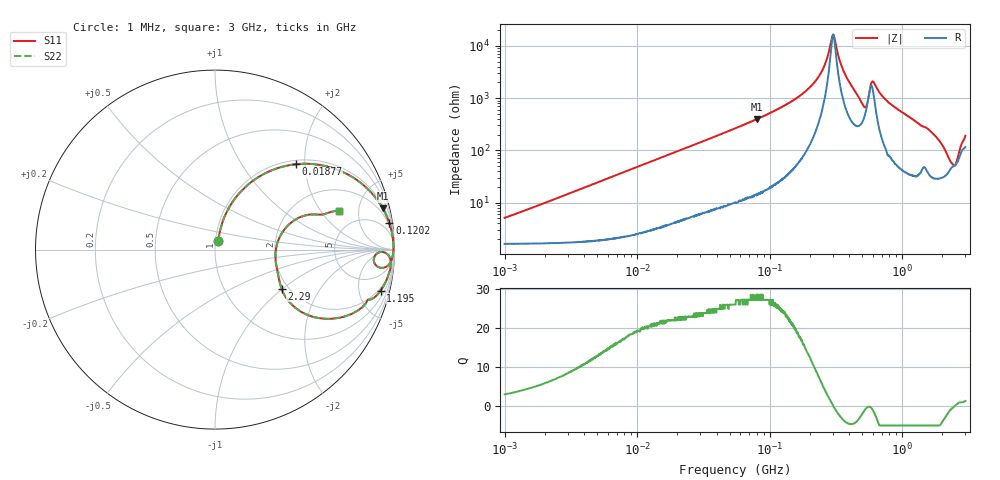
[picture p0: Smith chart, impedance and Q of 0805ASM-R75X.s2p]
!s-Parameter Generated by FASTRON Sdn. Bhd.
!FASTRON P/N : 0805ASM-R75X
!Keysight Technologies: E4991B_MY54100416_A.01.15
!Date: Fri Jun 19 14:53:31 2026
!Version  :Rev00  Fri Jun 19 14:53:31 2026
!Data & Calibration Information:
!Freq  S11  S21  S12  S22
!PortZ  Port1:50+j0  Port2:50+j0
!When reading reference impedance value at option line is always used.
! Remarks : This data is being provided solely for informational purposes.
# Hz S dB R 50
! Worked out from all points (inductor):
!   1601 points, 1 MHz to 3 GHz, reference 50 ohm
!   read as one part in series: L = 772 nH near 1.041 MHz
!   highest Q = 27.3 at 80.52 MHz (marker M1), where L = 792 nH
!   self-resonance near 301.7 MHz
!   S11 on the Smith chart (normalised r, x): 1 MHz: 1.03, +0.10; 18.77 MHz: 1.08, +1.80; 120.2 MHz: 2, +13; 1.195 GHz: 1.65, -7.86; 2.29 GHz: 1.84, -0.98; 3 GHz: 3.32, +3.02
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1000000  -26.00 68.7  -0.15 -2.7  -0.15 -2.7  -26.00 68.7
3804036  -14.90 74.2  -0.29 -10.3  -0.29 -10.3  -14.90 74.2
1.447069e7  -5.06 53.4  -1.90 -33.9  -1.90 -33.9  -5.06 53.4
1.877136e7  -3.69 46.6  -2.76 -40.8  -2.76 -40.8  -3.69 46.6
5.504702e7  -0.69 20.4  -9.13 -67.4  -9.13 -67.4  -0.69 20.4
8.051876e7  -0.34 13.9  -12.40 -74.0  -12.40 -74.0  -0.34 13.9
1.201581e8  -0.15 8.7  -16.40 -79.0  -16.40 -79.0  -0.15 8.7
2.083556e8  -0.06 3.2  -25.00 -81.7  -25.00 -81.7  -0.06 3.2
2.545267e8  -0.05 1.5  -31.60 -76.9  -31.60 -76.9  -0.05 1.5
3.017325e8  -0.05 0.0  -44.40 -1.9  -44.40 -1.9  -0.05 0.0
3.649251e8  -0.07 -1.8  -29.90 73.5  -29.90 73.5  -0.07 -1.8
5.051982e8  -0.61 -6.3  -18.00 54.3  -18.00 54.3  -0.61 -6.3
5.364635e8  -1.05 -3.5  -17.90 25.1  -17.90 25.1  -1.05 -3.5
6.018993e8  -0.28 -2.0  -26.60 46.0  -26.60 46.0  -0.28 -2.0
7.925923e8  -0.16 -6.8  -18.40 77.6  -18.40 77.6  -0.16 -6.8
1.194682e9  -0.44 -13.9  -12.40 71.4  -12.40 71.4  -0.44 -13.9
1.637435e9  -1.15 -21.9  -8.48 60.2  -8.48 60.2  -1.15 -21.9
1.960646e9  -2.61 -31.4  -5.46 46.3  -5.46 46.3  -2.61 -31.4
2.289646e9  -7.33 -30.4  -3.53 19.1  -3.53 19.1  -7.33 -30.4
2.505452e9  -9.35 1.5  -3.62 -0.8  -3.62 -0.8  -9.35 1.5
2.687267e9  -5.82 20.9  -5.15 -19.3  -5.15 -19.3  -5.82 20.9
3e9  -2.82 17.5  -8.43 -35.0  -8.43 -35.0  -2.82 17.5
